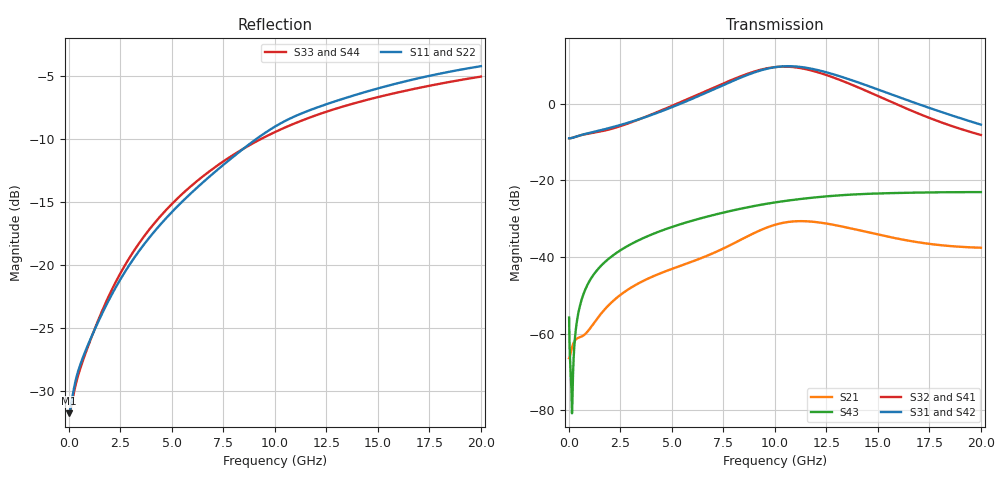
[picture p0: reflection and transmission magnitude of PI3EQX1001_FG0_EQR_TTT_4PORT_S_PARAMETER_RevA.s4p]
! NPort=4 DATA=2000 NOISE=0 GROUPDELAY=0 COMPLEX_DATAFORMAT=POLAR
! NumOfBlock=1 NumOfParam=0
! .MODEL Smodel S TSTONEFILE=PI3EQX1001_FG0_EQR_TTT_4PORT_S_PARAMETER_RevA.s4p TYPE=S
!  -- The above .MODEL line can be used for the S element in the netlist.
! The s parameter is extracted from the linear redriver, it is not bi-directional; only s(4,1)s(4,2) and s(3,1)s(3,2)
! should be the insertion loss
!Port definition:
!Port1 = input+
!Port2 = input¨C
!Port3 = output+
!Port4 = output-
# Hz S MA R  50
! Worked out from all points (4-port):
!   2000 points, 10 MHz to 20 GHz, reference 50 ohm
!   strongest paths, dB at 10 MHz, 5.01 GHz, 10.01 GHz, 15.01 GHz, 20 GHz:
!     S31: -9.0, -0.9, 9.5, 3.7, -5.5
!     S42: -9.0, -0.9, 9.5, 3.7, -5.5
!     S32: -9.0, -0.5, 9.6, 2.0, -8.1
!     S41: -9.0, -0.6, 9.5, 1.9, -8.2
!     S43: -55.8, -32.1, -25.7, -23.4, -23.1
!     S21: -66.4, -43.1, -31.6, -34.1, -37.6
!   lowest |S11| = -31.7 dB at 10 MHz (marker M1), VSWR 1.05, Z = 47.5 - j0.063 ohm
!   |S11| at or under -10 dB: start of sweep to 9.113 GHz
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1e7  0.0259 -178.5  0.0004902 2.7  3.669e-05 -0.2  4.787e-05 -0.1
     0.000479 2.9  0.02597 -178.7  4.577e-05 -0.2  5.994e-05 -0.1
     0.3546 -0.3  0.3545 179.7  0.02616 178.4  0.001616 -59.1
     0.3544 179.7  0.3544 -0.3  0.001626 -59.0  0.02613 178.4
7.6e9  0.2533 -106.1  0.01262 77.3  2.132e-05 -31.0  3.186e-05 -29.8
       0.01333 75.4  0.2513 -106.0  2.86e-05 -24.9  3.935e-05 -25.2
       1.801 -59.2  1.891 127.2  0.2607 -112.4  0.03861 53.9
       1.882 127.3  1.796 -59.2  0.03859 53.9  0.2604 -112.3
9.61e9  0.3373 -108.8  0.0233 57.2  1.916e-05 -27.6  3.419e-05 -34.2
        0.02425 55.6  0.3349 -108.8  3.174e-05 -26.4  3.716e-05 -24.0
        2.861 -115.0  2.898 71.1  0.3243 -115.3  0.04962 41.2
        2.881 71.2  2.853 -115.1  0.04961 41.1  0.3241 -115.3
1.128e10  0.3979 -113.6  0.02831 25.0  2.206e-05 -19.2  3.581e-05 -48.7
          0.02941 23.7  0.3949 -113.7  3.375e-05 -40.3  4.021e-05 -21.0
          3.015 -173.0  2.906 13.8  0.3726 -118.3  0.05741 29.6
          2.888 14.1  3.007 -173.0  0.05735 29.6  0.3723 -118.2
1.363e10  0.464 -118.8  0.02281 -7.7  3.088e-05 -37.5  3.002e-05 -74.5
          0.02383 -8.7  0.4602 -118.8  2.774e-05 -64.0  4.846e-05 -34.2
          2.073 117.6  1.82 -52.7  0.4318 -122.3  0.06523 13.3
          1.807 -52.3  2.067 117.6  0.06508 13.3  0.4317 -122.3
1.609e10  0.5278 -123.3  0.01621 -19.6  3.052e-05 -71.8  2.1e-05 -106.8
          0.01711 -20.9  0.5234 -123.3  1.783e-05 -92.1  4.518e-05 -58.3
          1.201 63.9  0.9371 -99.3  0.4848 -126.0  0.06879 -2.3
          0.9311 -98.7  1.197 63.9  0.06868 -2.3  0.4845 -126.0
2e10  0.6128 -130.1  0.01263 -16.1  1.805e-05 -142.3  1.586e-05 145.6
      0.01322 -19.0  0.6074 -130.2  1.097e-05 131.4  2.155e-05 -97.1
      0.5339 1.2  0.3914 -141.3  0.5572 -131.2  0.07037 -23.8
      0.3912 -140.4  0.5319 1.2  0.0703 -23.9  0.5571 -131.1
